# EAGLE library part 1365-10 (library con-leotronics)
DUAL ROW STRAIGHT HEADER 1364 SERIES. 1.27mm x 1.27mm. Without Fixing Post. SMT Source: http://www.leotronics.co.uk/Conexcon/Data%20Sheets/sec.%20A/1364ing.pdf
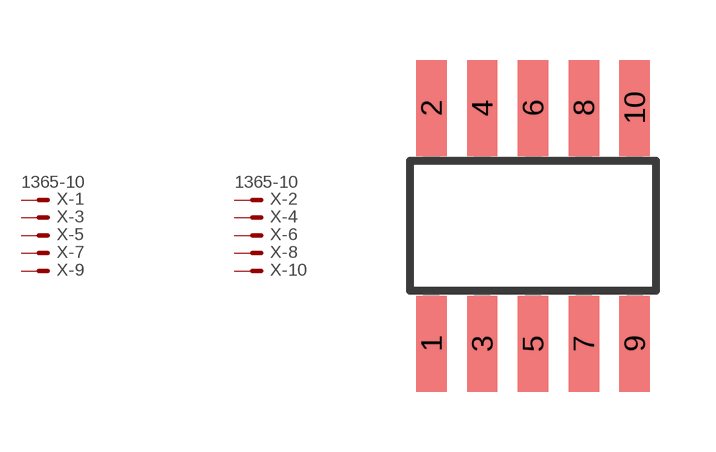
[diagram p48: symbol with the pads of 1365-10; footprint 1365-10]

Designator prefix X; gates -1=MVAL -2=MVAL -3=M -4=M -5=M -6=M -7=M -8=M -9=M -10=M

## 1365-10 (OC_FARNELL: unknown; OC_NEWARK: unknown)  [1365-10]
1  -1:S  pas
2  -2:S  pas
3  -3:S  pas
4  -4:S  pas
5  -5:S  pas
6  -6:S  pas
7  -7:S  pas
8  -8:S  pas
9  -9:S  pas
10  -10:S  pas

## Footprint 1365-10 (pad centres in mm)
DUAL ROW STRAIGHT HEADER 1364 SERIES. 1.27mm x 1.27mm. Without Fixing Post. SMT Source: http://www.leotronics.co.uk/Conexcon/Data%20Sheets/sec.%20A/1364ing.pdf
smd 0.76 x 2.4: 1 -2.54,-2.95; 2 -2.54,2.95; 3 -1.27,-2.95; 4 -1.27,2.95; 5 0,-2.95; 6 0,2.95; 7 1.27,-2.95; 8 1.27,2.95; 9 2.54,-2.95; 10 2.54,2.95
